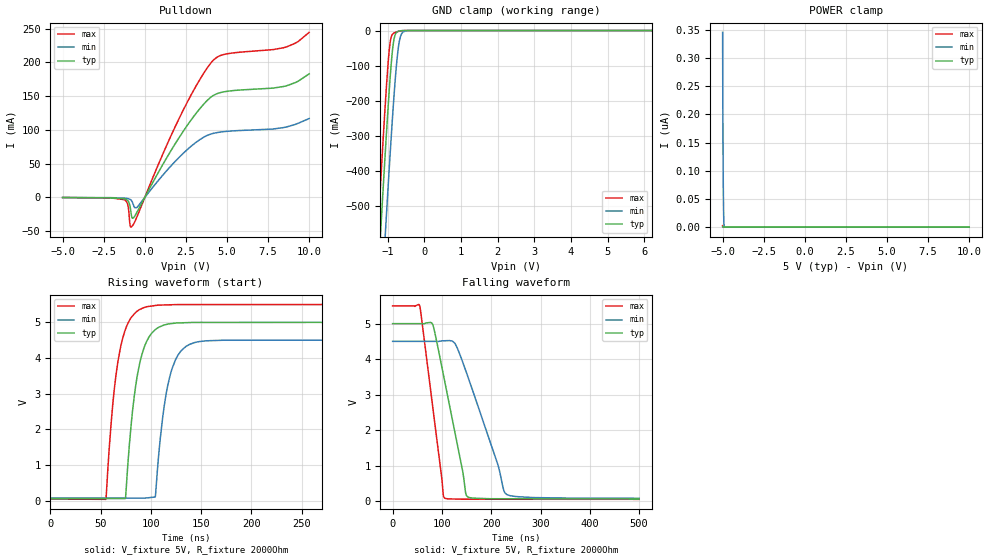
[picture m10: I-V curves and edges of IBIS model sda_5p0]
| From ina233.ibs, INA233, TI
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|   sda_5p0
[Model]   sda_5p0
Model_type   I/O_open_drain
Polarity   Non-Inverting
Vinl = 0.4
Vinh = 3.5
Vmeas = 2.5
Vref = 5.0
Cref = 2pF
Rref = 2000
|   typ   min   max
C_comp   1.140E-12   1.070E-12   1.244E-12
|C_comp_pull_down   1.365E-12   1.341E-12  1.375E-12
| Where Nom  PVT is Nominal Process, 5V, 25C
|   Fast PVT is Strong Process,  5.5V, -40C
|   Slow PVT is Weak Process,   4.5V, 125C
[Voltage Range]   5   4.5   5.5
[Temperature Range]   25   125   -40
[Pullup Reference]   5   4.5   5.5
[Pulldown Reference]   0   0   0
[Power Clamp Reference]   5   4.5   5.5
[GND Clamp Reference]   0   0   0
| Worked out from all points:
|   slope of the pulldown table from 0 to 0.75 V, typ, clamps not added: 22.2 ohm
|   GND clamp passes 1 mA (typ) near -0.66 V on its own axis
|   falling waveform, V_fixture 5V, R_fixture 2000Ohm: 20-80 % time 42.6ns typ, 65ns min, 29.8ns max; typ from 5 V to 0.056 V
|   rising waveform, V_fixture 5V, R_fixture 2000Ohm: 20-80 % time 13.1ns typ, 13.3ns min, 12.9ns max; typ from 0.056 V to 5 V
[Pulldown]
|   Voltage   I(typ)   I(min)   I(max)
-5V       -175.5uA   -103.8uA   -209.4uA
-1.25V    -2.156mA   -993.5uA   -3.281mA
-1.04V    -4.675mA   -1.674mA   -10.26mA
-890mV    -14.05mA   -3.009mA   -42.19mA
-830mV    -24.04mA   -4.18mA    -43.88mA
-755mV    -30.86mA   -6.999mA   -42.01mA
-500mV    -22.93mA   -15.27mA   -30.03mA
2.11V     89.43mA    59.83mA    118mA
4.15V     150.6mA    94.7mA     202.6mA
5.05V     157.2mA    97.93mA    212.8mA
8.575V    165mA      104mA      222.5mA
10V       182.9mA    116.8mA    244.4mA
[GND Clamp]
|   Voltage   I(typ)   I(min)   I(max)
-5V       -8.058A    -8.271A    -7.934A
-1.43V    -1.024A    -1.261A    -883mA
-1.25V    -685.5mA   -922.8mA   -543.1mA
-1.16V    -520mA     -756.6mA   -378.3mA
-1.07V    -359.5mA   -593.6mA   -221.2mA
-1.04V    -307.8mA   -540.1mA   -172.1mA
-950mV    -162.4mA   -384.1mA   -50.55mA
-830mV    -27.42mA   -192.9mA   -7.551mA
-710mV    -2.247mA   -51.07mA   -2.53mA
-620mV    -400uA     -9.712mA   -670uA
-410mV    -2.011uA   -80.92uA   -2.42uA
10V       0A         0A         0A
[POWER Clamp]
|   Voltage   I(typ)   I(min)   I(max)
-5V       803.9pA    345.5nA    2.612nA
-4.985V   401.9pA    191.4nA    1.306nA
-4.97V    0A         112.8nA    0A
-4.955V   0A         61.92nA    0A
-4.94V    0A         29.06nA    0A
-4.925V   0A         7.834nA    0A
-4.895V   0A         0A         0A
10V       0A         0A         0A
[Ramp]
R_load = 2000
|   typ   min   max
dV/dt_r   2.96628/1.31093e-08   2.65453/1.33348e-08   3.27147/1.29392e-08
dV/dt_f   2.96628/4.25837e-08   2.65453/6.50013e-08   3.27147/2.97029e-08
[Falling Waveform]
V_fixture = 5V
V_fixture_min = 4.5V
V_fixture_max = 5.5V
R_fixture = 2000Ohm
C_fixture = 0F
|   Time   V(typ)   V(min)   V(max)
0s        5V         4.5V       5.5V
55ns      5V         4.5V       5.498V
81.19ns   4.98V      4.5V       2.673V
102.7ns   3.579V     4.516V     177.3mV
105.1ns   3.411V     4.517V     87.07mV
126.6ns   1.917V     4.435V     55.81mV
149.8ns   154.1mV    3.617V     50.78mV
225.5ns   63.8mV     297.4mV    50.08mV
231.1ns   63.64mV    188.1mV    50.03mV
500ns     56.2mV     75.79mV    47.56mV
[Rising Waveform]
V_fixture = 5V
V_fixture_min = 4.5V
V_fixture_max = 5.5V
R_fixture = 2000Ohm
C_fixture = 0F
|   Time   V(typ)   V(min)   V(max)
0s        56.2mV     75.79mV    47.56mV
55.35ns   59.34mV    73.73mV    38.5mV
63.89ns   59.82mV    73.41mV    3.18V
74.71ns   60.44mV    73.01mV    4.798V
83.6ns    2.948V     72.68mV    5.237V
92.72ns   4.241V     72.34mV    5.41V
104.5ns   4.797V     125.1mV    5.472V
116.8ns   4.949V     3.228V     5.49V
138.5ns   4.994V     4.382V     5.498V
500ns     5V         4.5V       5.5V
